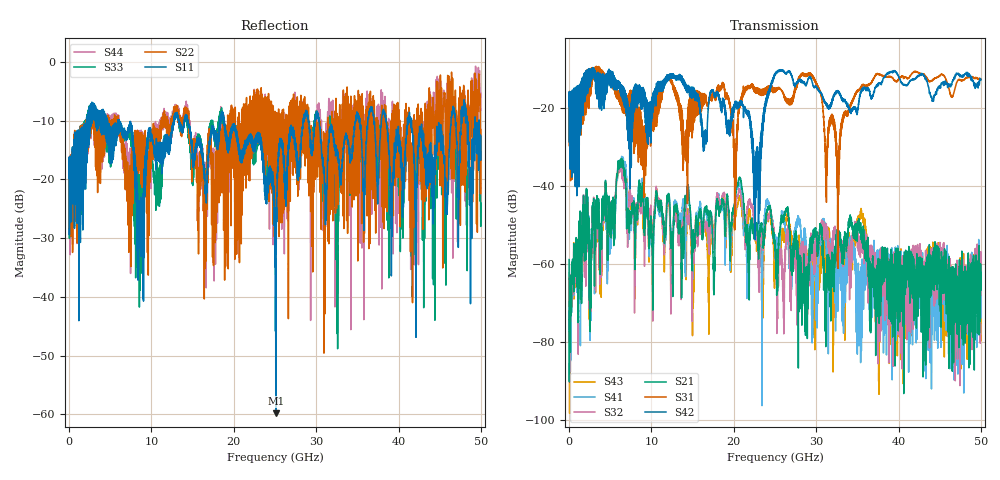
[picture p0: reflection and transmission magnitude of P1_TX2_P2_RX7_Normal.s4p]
!Keysight Technologies,N5225B,MY57041031,A.13.20.10
!Date: Friday, May 31, 2019 11:38:29
!Correction: S11(Full 4 Port(1,2,3,4))
!S12(Full 4 Port(1,2,3,4))
!S13(Full 4 Port(1,2,3,4))
!S14(Full 4 Port(1,2,3,4))
!S21(Full 4 Port(1,2,3,4))
!S22(Full 4 Port(1,2,3,4))
!S23(Full 4 Port(1,2,3,4))
!S24(Full 4 Port(1,2,3,4))
!S31(Full 4 Port(1,2,3,4))
!S32(Full 4 Port(1,2,3,4))
!S33(Full 4 Port(1,2,3,4))
!S34(Full 4 Port(1,2,3,4))
!S41(Full 4 Port(1,2,3,4))
!S42(Full 4 Port(1,2,3,4))
!S43(Full 4 Port(1,2,3,4))
!S44(Full 4 Port(1,2,3,4))
!S4P File: Measurements: <S11,S12,S13,S14>,
!<S21,S22,S23,S24>,
!<S31,S32,S33,S34>,
!<S41,S42,S43,S44>:
# Hz S  dB  R 50.0
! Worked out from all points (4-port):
!   5000 points, 10 MHz to 50 GHz, reference 50 ohm
!   strongest paths, dB at 10 MHz, 12.51 GHz, 25.01 GHz, 37.51 GHz, 50 GHz:
!     S42: -19.4, -12.2, -11.6, -13.9, -12.7
!     S31: -19.4, -13.0, -15.4, -11.1, -12.5
!     S21: -58.8, -53.1, -56.3, -68.4, -62.1
!     S32: -62.1, -55.1, -54.9, -69.0, -60.2
!     S41: -71.2, -53.7, -53.4, -60.9, -69.3
!     S43: -63.6, -58.9, -59.1, -68.8, -79.6
!   lowest |S11| = -59.8 dB at 25.1 GHz (marker M1), VSWR 1.00, Z = 49.9 + j0.0806 ohm
!   |S11| at or under -10 dB: 6.091 GHz to 12.71 GHz (6.616 GHz wide, 70.4 % of centre); 18.82 GHz to 28.43 GHz (9.605 GHz wide, 40.7 % of centre); 41.58 GHz to 46.38 GHz (4.809 GHz wide, 10.9 % of centre)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
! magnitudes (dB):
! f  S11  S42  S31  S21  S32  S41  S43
! 10 MHz  -19.8  -19.4  -19.4  -58.8  -62.1  -71.2  -63.6
! 6.35 GHz  -11.6  -16.6  -19.6  -33.4  -35.2  -33.1  -34.4
! 22.8 GHz  -13.5  -37.2  -15.2  -49.5  -51.4  -51.4  -54.4
! 25.1 GHz  -59.8  -11.1  -15.1  -57.2  -56.8  -54.2  -57.5
! 31.66 GHz  -11.8  -19.5  -24.5  -63.8  -62.9  -55.5  -55.1
! 32.64 GHz  -15.8  -15.5  -37.5  -53.3  -54.2  -65.7  -53.5
! 50 GHz  -12.6  -12.7  -12.5  -62.1  -60.2  -69.3  -79.6
